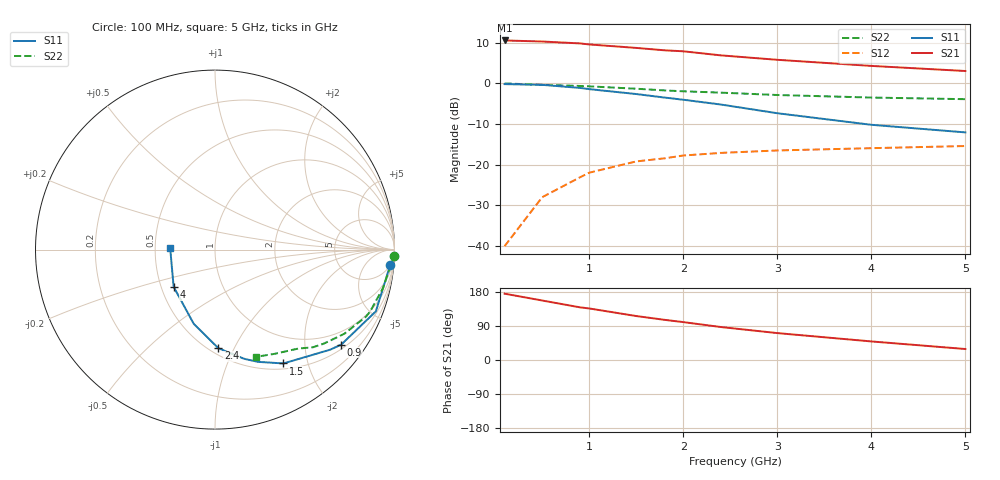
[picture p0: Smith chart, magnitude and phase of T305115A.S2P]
!AT-30511
!S and NOISE PARAMETERS at Vce=5V  Ic=1mA.  LAST UPDATED 06-23-94
# ghz s ma r 50
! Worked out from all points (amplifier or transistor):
!   11 points, 100 MHz to 5 GHz, reference 50 ohm
!   highest |S21| = 10.6 dB at 100 MHz (marker M1)
!   |S21| within 3 dB of that: start of sweep to 2.134 GHz
!   unconditionally stable (mu >= 1): 3.63 GHz to end of sweep
!   at 500 MHz: K = 0.17, MSG = 19.1 dB, |S12| = -28.0 dB
!   at 1.8 GHz: K = 0.56, MSG = 13.3 dB, |S12| = -18.4 dB
!   at 5 GHz: K = 1.19, MAG = 6.6 dB, |S12| = -15.4 dB
!   lowest NFmin = 0.30 dB at 500 MHz
!   S11 on the Smith chart (normalised r, x): 100 MHz: 5, -22; 900 MHz: 0.61, -2.87; 1.5 GHz: 0.58, -1.62; 2.4 GHz: 0.55, -0.87; 4 GHz: 0.58, -0.27; 5 GHz: 0.60, +0.01
0.1  0.98 -5.0  3.37 175.0  0.01 87.0  0.999 -2.0
0.5  0.96 -21.0  3.27 157.0  0.04 74.0  0.96 -13.0
0.9  0.88 -37.0  3.1 139.0  0.07 64.0  0.93 -22.0
1  0.85 -41.0  3.01 136.0  0.08 62.0  0.92 -24.0
1.5  0.74 -59.0  2.73 116.0  0.11 51.0  0.86 -33.0
1.8  0.67 -69.0  2.55 106.0  0.12 45.0  0.82 -38.0
2  0.63 -75.0  2.48 100.0  0.13 42.0  0.8 -41.0
2.4  0.55 -88.0  2.21 87.0  0.14 37.0  0.77 -45.0
3  0.43 -106.0  1.95 71.0  0.15 31.0  0.72 -50.0
4  0.31 -138.0  1.64 49.0  0.16 23.0  0.67 -60.0
5  0.25 178.0  1.42 29.0  0.17 20.0  0.64 -69.0
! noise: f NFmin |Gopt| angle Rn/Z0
0.5  0.3  0.96  10  1.49
0.9  0.4  0.92  19  1.33
1.8  0.9  0.83  43  0.98
2.4  1.3  0.76  60  0.74
